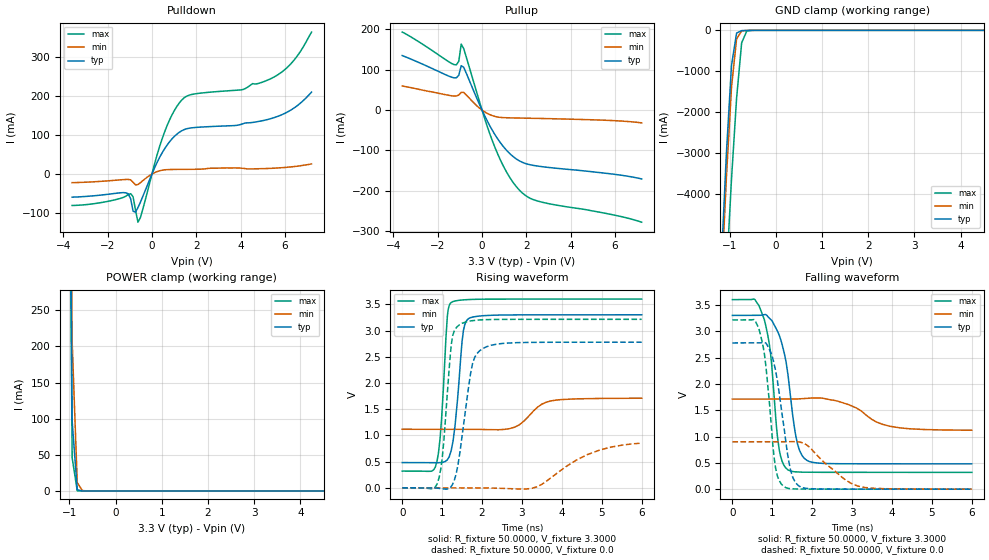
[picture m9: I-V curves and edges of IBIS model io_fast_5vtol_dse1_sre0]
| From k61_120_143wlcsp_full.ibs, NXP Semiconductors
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[Model]  io_fast_5vtol_dse1_sre0
|   Model io_fast_5vtol_dse1_sre0
| Library cells for typ/min/max conditions are connected as defined below:
|  pad - External Pad
|  ipp_do - Core Input
|  ipp_obe - Output Buffer Enable
|  esd_boost - vdd_s_3v
|  esd_bus - vdd_s_3v
|  ipp_ame - vss_s_lv
|  ipp_dse - vdd_s_lv
|  ipp_ina40a_5vtol - NC
|  ipp_ina40b_5vtol - NC
|  ipp_ina_5vtol - NC
|  ipp_ina_mux_3v - NC
|  ipp_ind - NC
|  ipp_ind_3v - NC
|  ipp_pue - vss_s_lv
|  ipp_sre - vss_s_lv
|  tie_3v - vdd_s_3v
|  tie_hi - vdd_s_lv
|  vbuf_3v - vdd_s_3v
|  vdd_bulk_lv - vdd_s_lv
|  vdd_s_3v - vdd_s_3v
|  vdd_s_lv - vdd_s_lv
|  vss_bulk - vss_s_3v
|  vss_s_3v - vss_s_3v
|  vss_s_lv - vss_s_lv
| All other pins connected to ground
Model_type I/O
Polarity   Non-Inverting
Enable   Active-High
Vinl =   1.1550V
Vinh =   2.3100V
Vmeas =  1.6500V
Cref =   25.0000pF
Rref =   50.0000
Vref =   0.0V
C_comp   4.6092pF   4.5386pF   4.8302pF
[Temperature Range]   25.0000   0.1250k   -40.0000
[Voltage Range]   3.3000V   1.7100V   3.6000V
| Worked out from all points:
|   slope of the pulldown table from 0 to 0.495 V, typ, clamps not added: 8.59 ohm
|   slope of the pullup table from 0 to 0.495 V, typ, clamps not added: 9.33 ohm
|   GND clamp passes 1 mA (typ) near -0.54 V on its own axis
|   POWER clamp passes 1 mA (typ) near -0.79 V on its own axis
|   rising waveform, R_fixture 50.0000, V_fixture 3.3000: 20-80 % time 194ps typ, 498ps min, 150ps max; typ from 0.481 V to 3.3 V
|   rising waveform, R_fixture 50.0000, V_fixture 0.0: 20-80 % time 303ps typ, 1.12ns min, 197ps max; typ from 0 V to 2.78 V
|   falling waveform, R_fixture 50.0000, V_fixture 3.3000: 20-80 % time 332ps typ, 783ps min, 251ps max; typ from 3.3 V to 0.482 V
|   falling waveform, R_fixture 50.0000, V_fixture 0.0: 20-80 % time 317ps typ, 797ps min, 239ps max; typ from 2.78 V to 0 V
[Pulldown]
|Voltage   I(typ)   I(min)   I(max)
-3.6V     -59.22mA   -21.99mA   -80.5mA
-1.29V    -47.58mA   -14.27mA   -59.74mA
-960mV    -63.34mA   -14.81mA   -50.29mA
-850mV    -95.19mA   -20.91mA   -58.11mA
-630mV    -85.86mA   -26.77mA   -123.3mA
470mV     55.27mA    9.989mA    91.83mA
910mV     90.4mA     11.72mA    152.1mA
1.35V     111mA      11.98mA    189.9mA
4.1V      128.8mA    14.7mA     216.5mA
5.42V     142.9mA    14.8mA     246mA
6.41V     169.2mA    19.2mA     291.7mA
7.2V      210mA      26.1mA     363.7mA
[Pullup]
|Voltage   I(typ)   I(min)   I(max)
-3.6V     135.3mA    59.8mA     193.5mA
-1.27V    80.13mA    34.99mA    113mA
-1.16V    80.16mA    35.07mA    112.2mA
-1.05V    86.44mA    37.35mA    121mA
-940mV    110.2mA    44.17mA    163.6mA
-830mV    106.4mA    44mA       152.9mA
160mV     -18.66mA   -5.726mA   -28.08mA
710mV     -71.72mA   -17.2mA    -109.3mA
1.26V     -108.3mA   -19.14mA   -167.8mA
1.92V     -131.7mA   -19.93mA   -210.1mA
2.69V     -140.1mA   -20.72mA   -228.1mA
7.2V      -170.7mA   -31.6mA    -277.9mA
[GND_clamp]
|Voltage   I(typ)   I(min)   I(max)
-3.6V     -73.34A    -73.38A    -74.77A
-1.18V    -5.66A     -6.204A    -8.642A
-1.07V    -2.998A    -3.591A    -5.955A
-960mV    -859.3mA   -1.396A    -3.637A
-850mV    -67.61mA   -209.6mA   -1.663A
-740mV    -7.668mA   -15.82mA   -304.8mA
-630mV    -2.587mA   -2.146mA   -18.83mA
-520mV    -662.1uA   -523uA     -1.741mA
7.2V      0A         0A         0A
[POWER_clamp]
|Voltage   I(typ)   I(min)   I(max)
-3.6V     45.85A     45.45A     46.17A
-1.05V    1.004A     1.14A      941.6mA
-940mV    96.57mA    206.1mA    45.73mA
-830mV    1.646mA    11.48mA    218.1uA
-720mV    22.84uA    474.3uA    919.1nA
-610mV    316.6nA    19.24uA    4.178nA
7.2V      0A         0A         0A
[Ramp]
| variable   typ   min   max
dV/dt_r  1.6661/0.3026n   0.5118/1.1218n   1.9282/0.1974n
dV/dt_f  1.6910/0.3315n   0.3541/0.7833n   1.9683/0.2510n
R_load = 50.0000
[Rising Waveform]
R_fixture= 50.0000
V_fixture= 3.3000
V_fixture_min= 1.7100
V_fixture_max= 3.6000
|time   V(typ)   V(min)   V(max)
0s        481.4mV    1.117V     319.2mV
869.4ps   478.5mV    1.117V     498.7mV
984.4ps   484mV      1.117V     1.301V
1.123ns   529.5mV    1.117V     3.221V
1.232ns   730.8mV    1.117V     3.538V
1.535ns   3.004V     1.117V     3.585V
1.653ns   3.223V     1.117V     3.59V
2.816ns   3.298V     1.156V     3.599V
3.718ns   3.299V     1.656V     3.6V
6ns       3.3V       1.709V     3.6V
[Rising Waveform]
R_fixture= 50.0000
V_fixture= 0.0
V_fixture_min= 0.0
V_fixture_max= 0.0
|time   V(typ)   V(min)   V(max)
0s        310.4pV    53.91nV    167.4pV
883.2ps   -6.264mV   -1.012uV   91.17mV
1.002ns   -17.66mV   1.21uV     566.2mV
1.229ns   30.2mV     -25.9uV    2.734V
1.43ns    598mV      192.7uV    3.107V
1.762ns   2.37V      331.7uV    3.188V
2.01ns    2.652V     -380uV     3.205V
3.251ns   2.774V     -8.832mV   3.213V
4.648ns   2.777V     636mV      3.214V
6ns       2.777V     853mV      3.214V
[Falling Waveform]
R_fixture= 50.0000
V_fixture= 3.3000
V_fixture_min= 1.7100
V_fixture_max= 3.6000
|time   V(typ)   V(min)   V(max)
0s        3.3V       1.71V      3.6V
543.4ps   3.3V       1.71V      3.61V
800.6ps   3.315V     1.71V      3.22V
951.8ps   3.23V      1.71V      2.618V
1.168ns   2.937V     1.71V      774.1mV
1.394ns   2.171V     1.71V      365.3mV
1.635ns   853.2mV    1.714V     326.3mV
1.867ns   547.3mV    1.726V     321.4mV
3.961ns   481.9mV    1.193V     319.5mV
6ns       481.7mV    1.12V      319.4mV
[Falling Waveform]
R_fixture= 50.0000
V_fixture= 0.0
V_fixture_min= 0.0
V_fixture_max= 0.0
|time   V(typ)   V(min)   V(max)
0s        2.777V     899.5mV    3.214V
543.3ps   2.777V     899.5mV    3.221V
663.5ps   2.777V     899.5mV    3.049V
824.9ps   2.779V     899.5mV    2.442V
1.083ns   2.253V     899.1mV    403.1mV
1.276ns   1.268V     899.8mV    58.03mV
1.46ns    359.1mV    902.5mV    9.248mV
1.719ns   38.82mV    888.4mV    2.02mV
3.137ns   422.9uV    60.93mV    262.9uV
6ns       233.4uV    312.3uV    181.6uV
